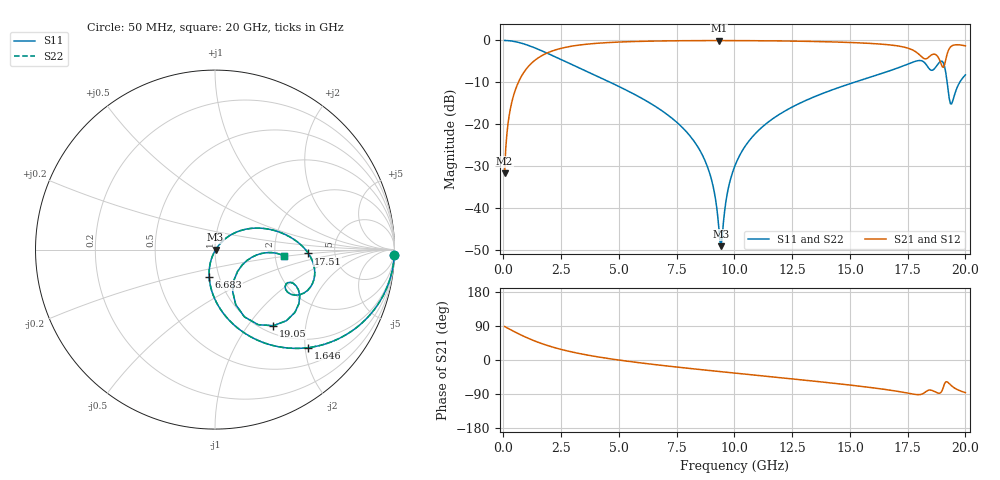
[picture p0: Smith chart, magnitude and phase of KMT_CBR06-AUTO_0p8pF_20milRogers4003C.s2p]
! Data measured by Modelithics Inc. support@modelithics.com 813-866-6335
! KEMET CBR06-AUTO 0.8pF, Pad Width= 0.851mm, Pad Length= 0.64mm, Pad Gap= 0.62mm, 20mil Rogers 4003C substrate Data, January 2022
# hz S ma R 50
! 2 Port Network Data from SP1.SP block
! freq  magS11  angS11  magS21  angS21  magS12  angS12  magS22  angS22
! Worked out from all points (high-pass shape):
!   401 points, 50 MHz to 20 GHz, reference 50 ohm
!   highest |S21| = -0.03 dB at 9.327 GHz (marker M1); lowest = -31.8 dB at 50 MHz (marker M2)
!   |S21| within 3 dB of the highest: 1.877 GHz to 17.93 GHz (16.05 GHz wide, 162 % of centre); 19.22 GHz to end of sweep
!   lowest |S11| = -49.2 dB at 9.427 GHz (marker M3), VSWR 1.01, Z = 50.3 - j0.119 ohm
!   |S11| at or under -10 dB: 4.619 GHz to 15.19 GHz (10.57 GHz wide, 107 % of centre); 19.21 GHz to 19.76 GHz (546.4 MHz wide, 2.8 % of centre)
!   |S22| runs from -49.2 to 0.0 dB; largest |S21 - S12| = 0
!   S11 on the Smith chart (normalised r, x): 50 MHz: 1, -70; 1.646 GHz: 0.82, -2.07; 6.683 GHz: 0.90, -0.28; 17.51 GHz: 3.16, -0.18; 19.05 GHz: 1.13, -1.34; 20 GHz: 2.24, -0.19
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5e7  0.9997 -1.6  0.02568 88.4  0.02568 88.4  0.9997 -1.6
2.495e8  0.9918 -8.1  0.1272 81.8  0.1272 81.8  0.9918 -8.1
5.4875e8  0.9621 -17.6  0.272 72.4  0.272 72.4  0.9621 -17.6
1.646e9  0.7547 -46.4  0.6547 43.5  0.6547 43.5  0.7547 -46.4
3.391625e9  0.4544 -73.9  0.8886 15.8  0.8886 15.8  0.4544 -73.9
6.683375e9  0.1557 -102.0  0.9847 -13.1  0.9847 -13.1  0.1557 -102.0
6.73325e9  0.1525 -102.3  0.9852 -13.4  0.9852 -13.4  0.1525 -102.3
8.6285e9  0.04182 -111.5  0.9956 -25.9  0.9956 -25.9  0.04182 -111.5
9.077375e9  0.018 -108.1  0.9962 -28.7  0.9962 -28.7  0.018 -108.1
9.32675e9  0.005678 -83.7  0.9963 -30.3  0.9963 -30.3  0.005678 -83.7
9.4265e9  0.003468 -20.0  0.9963 -30.9  0.9963 -30.9  0.003468 -20.0
9.72575e9  0.01659 45.1  0.9961 -32.8  0.9961 -32.8  0.01659 45.1
1.0025e10  0.03187 49.0  0.9956 -34.6  0.9956 -34.6  0.03187 49.0
1.117212e10  0.09061 45.9  0.9916 -41.6  0.9916 -41.6  0.09061 45.9
1.336662e10  0.2069 33.4  0.973 -55.3  0.973 -55.3  0.2069 33.4
1.670825e10  0.4323 8.6  0.8854 -79.3  0.8854 -79.3  0.4323 8.6
1.750625e10  0.5208 -2.3  0.8094 -87.4  0.8094 -87.4  0.5208 -2.3
1.885288e10  0.5386 -28.8  0.6087 -87.7  0.6087 -87.7  0.5386 -28.8
1.905238e10  0.5348 -52.5  0.4766 -70.2  0.4766 -70.2  0.5348 -52.5
1.9202e10  0.3279 -69.4  0.6763 -57.4  0.6763 -57.4  0.3279 -69.4
1.94015e10  0.1741 -29.5  0.8574 -68.1  0.8574 -68.1  0.1741 -29.5
2e10  0.3869 -5.3  0.8617 -86.2  0.8617 -86.2  0.3869 -5.3
